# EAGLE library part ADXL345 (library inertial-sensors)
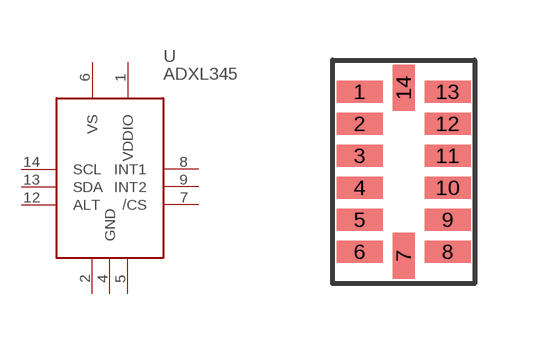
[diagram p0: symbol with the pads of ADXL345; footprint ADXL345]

Designator prefix U

## ADXL345  [ADXL345]
1  VDDIO
2  GND1
4  GND
5  GND3
6  VS
7  /CS
8  INT1
9  INT2
12  ALT
13  SDA
14  SCL

## Footprint ADXL345 (pad centres in mm)
smd 1.145 x 0.55: 1 -1.1,2; 2 -1.1,1.2; 3 -1.1,0.4; 4 -1.1,-0.4; 5 -1.1,-1.2; 6 -1.1,-2; 8 1.1,-2; 9 1.1,-1.2; 10 1.1,-0.4; 11 1.1,0.4; 12 1.1,1.2; 13 1.1,2
smd 0.55 x 1.145: 7 0,-2.1; 14 0,2.1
